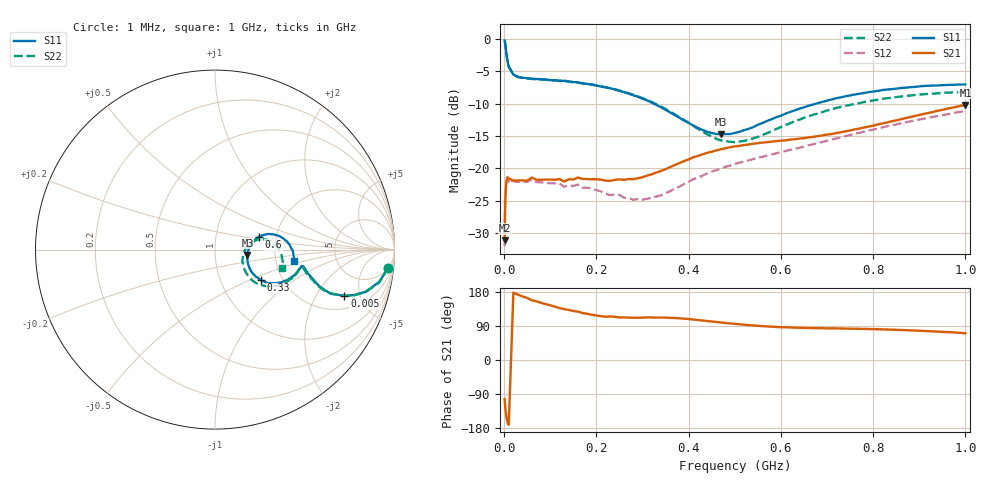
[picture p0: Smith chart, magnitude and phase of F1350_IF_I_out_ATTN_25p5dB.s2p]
! S-parameters for IF_I+ & IF_I- IDT F1350 DPD Demodulator
! Date Measured:  2015-11-25  RGG
!  Port 1 = Pin 19 = IF_I+
!  Port 2 = Pin 20 = IF_I-
! State: 25.5 dB attenuation (Gain = Gmax - 25.5 dB)
! IF Frequency:  1 MHz to 1000 MHz
! RF_INX, RF_INY, IF_Q+, and IF_Q- terminated
! 2300 MHz, 0 dBm signal applied to LO_IN
! Vcc = +5.00 Volts  Icc = approx 275 mA
! NOTES:  The device was measured on a custom printed circuit evaluation board with individual 50 ohm
!  microstrip lines to the RF and LO pins. The IF outputs are normally connected to balun
!  transformers, which convert the balanced IF output signals to single ended (SE) 50 ohm signals
!  for normal test purposes. For these measurements, to measure the IFI+ and IFI- output SE s-parameters,
!  the chokes associated with the IFI+ and IFI- outputs were removed and a pair of pigtailed
!  50 ohm coaxial lines were soldered to the PCB at these points. 5.00 volt bias was provided
!  to these pins via external bias tees. Data was collected using a calibrated vector
!  network analyzer.  The pigtailed 50 ohm coaxial lines were de-embedded using reference
!  plane extensions. 100 ohm microstrip lines of length 386 mils and 218 mils for the IF_I+ and IF_I-
!  signals, respectively, were de-embedded using Agilent ADS, yielding the reference plane at the IC edge.
!  Only IFI+ and IFI- outputs were measured. IF_Q+ and IF_Q- should be identical.
!  This data is single-ended relative to ports IF_I+ and IF_I- (reference impedance = 50 ohms)
!  Common mode or differential S-parameters may be extracted from this data with a linear simulator.
# mhz S db R 50
! freq  dbS11  angS11  dbS21  angS21  dbS12  angS12  dbS22  angS22
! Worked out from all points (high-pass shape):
!   109 points, 1 MHz to 1 GHz, reference 50 ohm
!   highest |S21| = -10.21 dB at 1 GHz (marker M1); lowest = -31.1 dB at 1 MHz (marker M2)
!   |S21| within 3 dB of the highest: 811 MHz to end of sweep
!   lowest |S11| = -14.7 dB at 470 MHz (marker M3), VSWR 1.45, Z = 71.9 - j4.42 ohm
!   |S11| at or under -10 dB: 324 MHz to 676.9 MHz (352.8 MHz wide, 70.5 % of centre)
!   |S22| runs from -16.0 to -0.3 dB; largest |S21 - S12| = 0.065
!   S11 on the Smith chart (normalised r, x): 1 MHz: 5, -18; 5 MHz: 2.86, -3.57; 330 MHz: 1.56, -0.59; 600 MHz: 1.62, +0.25; 1 GHz: 2.53, -0.40
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1  -0.25 -5.9  -31.09 -103.1  -32.02 -108.0  -0.26 -6.0
2  -0.60 -11.0  -26.34 -119.8  -25.70 -119.3  -0.61 -11.5
3  -1.15 -15.5  -24.00 -132.8  -24.14 -134.1  -1.19 -15.5
4  -1.75 -18.0  -22.78 -141.4  -22.62 -142.4  -1.74 -18.1
5  -2.32 -19.7  -21.97 -150.6  -22.19 -150.1  -2.37 -19.7
7  -3.22 -20.9  -21.36 -161.8  -21.99 -163.2  -3.43 -20.8
10  -4.28 -19.2  -21.57 -171.3  -21.67 -171.4  -4.32 -19.4
20  -5.51 -14.1  -21.87 177.6  -22.00 178.5  -5.56 -14.5
60  -6.16 -10.8  -21.43 157.5  -21.71 158.7  -6.20 -11.2
130  -6.49 -15.9  -22.04 134.0  -22.85 136.9  -6.47 -16.7
160  -6.74 -18.9  -21.42 127.7  -22.50 129.4  -6.75 -20.3
170  -6.86 -19.6  -21.63 123.9  -23.00 125.7  -6.88 -21.0
280  -8.71 -30.6  -21.67 111.4  -24.85 114.8  -8.63 -33.6
330  -10.20 -33.5  -20.65 111.9  -24.36 122.4  -10.10 -38.3
340  -10.56 -33.6  -20.39 111.8  -24.17 122.8  -10.45 -39.0
420  -13.75 -24.9  -18.08 105.5  -21.45 123.9  -13.91 -34.6
470  -14.74 -9.3  -17.04 98.9  -20.04 119.3  -15.69 -21.3
510  -14.36 3.3  -16.53 94.5  -19.11 115.7  -15.86 -7.8
600  -11.87 16.3  -15.73 86.7  -17.50 109.1  -13.62 11.2
670  -10.14 16.3  -15.14 84.2  -16.27 104.7  -11.72 13.1
840  -7.77 5.2  -12.73 80.1  -13.35 92.6  -9.09 1.1
1000  -7.04 -8.2  -10.21 70.7  -11.14 78.5  -8.20 -15.1
